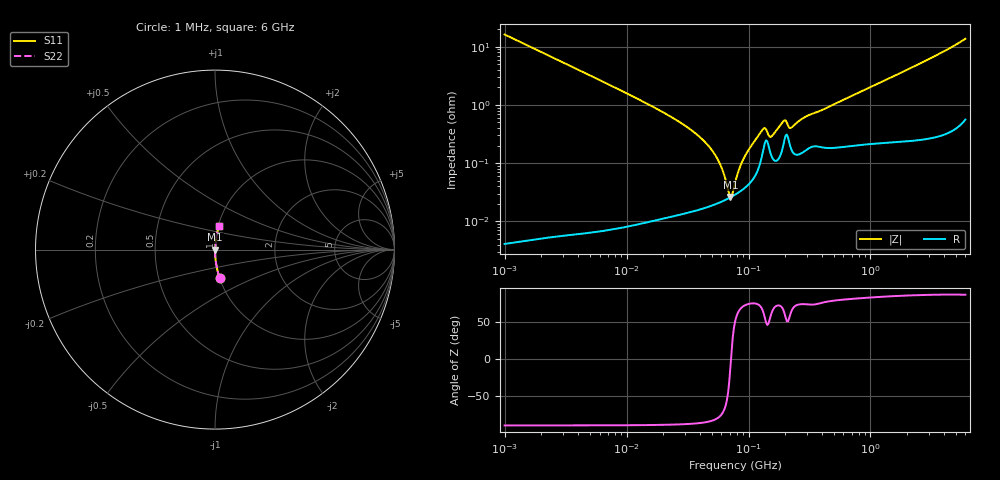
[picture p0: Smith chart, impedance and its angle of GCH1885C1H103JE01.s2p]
!Murata Part Number: GCH1885C1H103JE01
!These Parameters are Measured in Series Mode Connection
!Data Generated on Jun 19, 2026
!  o--ll--o
!Port1  Port2
!  o------o
!Operation Temp=25[degC], DC Bias Voltage=0[V]
!Freq. Start=1000[kHz] Stop=6[GHz] 401[Steps]
# Hz S RI R 50
!Freq.(Hz) S11(Real) S11(Imag) S21(Real) S21(Imag) S12(Real) S12(Imag) S22(Real) S22(Imag)
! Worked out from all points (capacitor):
!   401 points, 1 MHz to 6 GHz, reference 50 ohm
!   read as one part in series: C = 9.83 nF near 1.044 MHz
!   lowest |Z| = 26.4 mohm at 71.01 MHz (marker M1)
!   series resonance near 71.79 MHz, so ESL is about 500 pH
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1000000  0.0256 -0.1577  0.9744 0.1577  0.9744 0.1577  0.0256 -0.1577
4293785  0.00147 -0.0375  0.9985 0.0375  0.9985 0.0375  0.00147 -0.0375
1.843659e7  0.000175 -0.00818  0.9998 0.00818  0.9998 0.00818  0.000175 -0.00818
3.245342e7  0.000158 -0.00396  0.9998 0.00396  0.9998 0.00396  0.000158 -0.00396
4.697123e7  0.000182 -0.00198  0.9998 0.00198  0.9998 0.00198  0.000182 -0.00198
5.838291e7  0.000214 -0.000947  0.9998 0.000947  0.9998 0.000947  0.000214 -0.000947
6.23192e7  0.000226 -0.000647  0.9998 0.000647  0.9998 0.000647  0.000226 -0.000647
6.798347e7  0.000247 -0.000249  0.9998 0.000249  0.9998 0.000249  0.000247 -0.000249
7.100585e7  0.000259 -5.03e-05  0.9997 5.03e-05  0.9997 5.03e-05  0.000259 -5.03e-05
7.416259e7  0.000272 0.00015  0.9997 -0.00015  0.9997 -0.00015  0.000272 0.00015
7.745967e7  0.000287 0.000352  0.9997 -0.000352  0.9997 -0.000352  0.000287 0.000352
8.450008e7  0.000323 0.000765  0.9997 -0.000765  0.9997 -0.000765  0.000323 0.000765
9.218041e7  0.000371 0.0012  0.9996 -0.0012  0.9996 -0.0012  0.000371 0.0012
1.305463e8  0.00152 0.00346  0.9985 -0.00346  0.9985 -0.00346  0.00152 0.00346
1.363501e8  0.00226 0.00331  0.9977 -0.00331  0.9977 -0.00331  0.00226 0.00331
1.487431e8  0.0017 0.00228  0.9983 -0.00228  0.9983 -0.00228  0.0017 0.00228
1.553559e8  0.00128 0.00262  0.9987 -0.00262  0.9987 -0.00262  0.00128 0.00262
1.930997e8  0.00208 0.00483  0.9979 -0.00483  0.9979 -0.00483  0.00208 0.00483
2.248532e8  0.00171 0.0037  0.9983 -0.0037  0.9983 -0.0037  0.00171 0.0037
3.325952e8  0.00196 0.00676  0.998 -0.00676  0.998 -0.00676  0.00196 0.00676
1.428092e9  0.00306 0.0284  0.9969 -0.0284  0.9969 -0.0284  0.00306 0.0284
6e9  0.0236 0.1328  0.9764 -0.1328  0.9764 -0.1328  0.0236 0.1328
